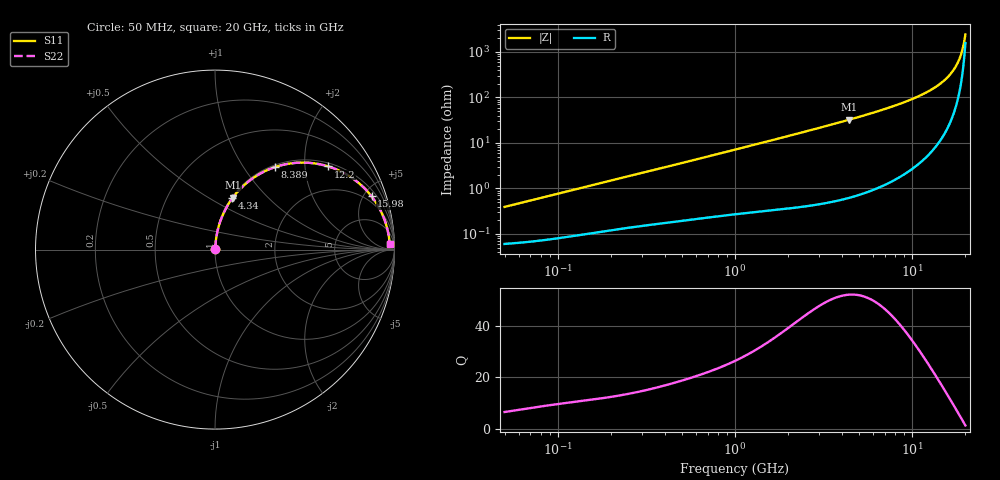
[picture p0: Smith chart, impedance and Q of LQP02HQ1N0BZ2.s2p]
!Murata Part Number: LQP02HQ1N0BZ2
!These Parameters are Measured in Series Mode Connection
!  o--[Z]--o
!Port1  Port2
!  o-------o
!Freq. Start=50[MHz] Stop=20[GHz], 401[Steps]
# Hz S RI R 50
!Freq.(Hz) S11(Real) S11(Imag) S21(Real) S21(Imag) S12(Real) S12(Imag) S22(Real) S22(Imag)
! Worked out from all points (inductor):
!   401 points, 50 MHz to 20 GHz, reference 50 ohm
!   read as one part in series: L = 1.23 nH near 51.52 MHz
!   highest Q = 52.2 at 4.406 GHz (marker M1), where L = 1.17 nH
!   S11 on the Smith chart (normalised r, x): 50 MHz: 1.00, +0.01; 4.34 GHz: 1.01, +0.64; 8.389 GHz: 1.03, +1.41; 12.2 GHz: 1.10, +2.64; 15.98 GHz: 1.45, +5.69; 20 GHz: 32, +37
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5e7  0.000617 0.00387  0.9994 -0.00387  0.9994 -0.00387  0.000617 0.00387
1.364002e8  0.00107 0.0103  0.9989 -0.0103  0.9989 -0.0103  0.00107 0.0103
3.721004e8  0.0024 0.027  0.9976 -0.027  0.9976 -0.027  0.0024 0.027
1e9  0.00768 0.0704  0.9923 -0.0704  0.9923 -0.0704  0.00768 0.0704
1.714689e9  0.0178 0.1189  0.9822 -0.1189  0.9822 -0.1189  0.0178 0.1189
2.728004e9  0.0403 0.1861  0.9597 -0.1861  0.9597 -0.1861  0.0403 0.1861
4.34015e9  0.0963 0.2856  0.9037 -0.2856  0.9037 -0.2856  0.0963 0.2856
4.405649e9  0.0991 0.2894  0.9009 -0.2894  0.9009 -0.2894  0.0991 0.2894
5.856089e9  0.1709 0.3666  0.8291 -0.3666  0.8291 -0.3666  0.1709 0.3666
7.442007e9  0.269 0.4325  0.731 -0.4325  0.731 -0.4325  0.269 0.4325
8.389408e9  0.3358 0.4603  0.6642 -0.4603  0.6642 -0.4603  0.3358 0.4603
1.034674e10  0.486 0.4849  0.514 -0.4849  0.514 -0.4849  0.486 0.4849
1.220001e10  0.6314 0.4633  0.3686 -0.4633  0.3686 -0.4633  0.6314 0.4633
1.417136e10  0.7714 0.3939  0.2286 -0.3939  0.2286 -0.3939  0.7714 0.3939
1.504638e10  0.8243 0.35  0.1757 -0.35  0.1757 -0.35  0.8243 0.35
1.597544e10  0.8723 0.2966  0.1277 -0.2966  0.1277 -0.2966  0.8723 0.2966
1.721783e10  0.9222 0.2176  0.0778 -0.2176  0.0778 -0.2176  0.9222 0.2176
1.774144e10  0.9381 0.1826  0.0619 -0.1826  0.0619 -0.1826  0.9381 0.1826
1.828096e10  0.9514 0.1461  0.0486 -0.1461  0.0486 -0.1461  0.9514 0.1461
1.88369e10  0.9617 0.1083  0.0383 -0.1083  0.0383 -0.1083  0.9617 0.1083
1.970266e10  0.9715 0.0498  0.0285 -0.0498  0.0285 -0.0498  0.9715 0.0498
2e10  0.9732 0.03  0.0268 -0.03  0.0268 -0.03  0.9732 0.03
